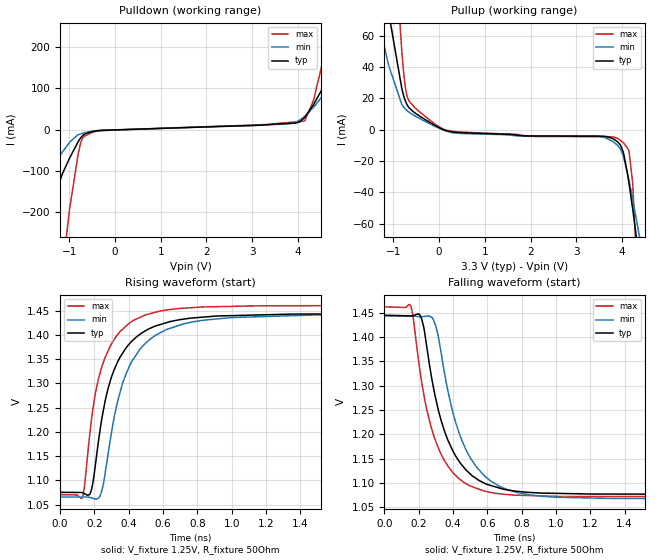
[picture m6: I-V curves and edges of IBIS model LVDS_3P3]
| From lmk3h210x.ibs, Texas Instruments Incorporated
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[Model]   LVDS_3P3
Model_type   Output
Polarity   Non-Inverting
Vmeas = 1.25
Vref = 1.25
Cref = 2pF
Rref = 50
|   typ   min   max
C_comp   2.5pF   2pF   3pF
[Voltage Range]   3.3   3.135   3.465
[Temperature Range]   45   125   -40
[Pullup Reference]   3.3   3.135   3.465
[Pulldown Reference]   -0   -0   0
[Power Clamp Reference]   3.3   3.135   3.465
[GND Clamp Reference]   0   0   0
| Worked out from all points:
|   slope of the pulldown table from 0 to 0.495 V, typ, clamps not added: 277 ohm
|   slope of the pullup table from 0 to 0.495 V, typ, clamps not added: 155 ohm
|   falling waveform, V_fixture 1.25V, R_fixture 50Ohm: 20-80 % time 175ps typ, 189ps min, 158ps max; typ from 1.45 V to 1.08 V
|   rising waveform, V_fixture 1.25V, R_fixture 50Ohm: 20-80 % time 169ps typ, 187ps min, 145ps max; typ from 1.08 V to 1.45 V
[Pulldown]
|   Voltage   I(typ)   I(min)   I(max)
-3.3V     -904.1mA   -523.3mA   -2.736A
-2.181V   -450.8mA   -243.4mA   -1.464A
-1.973V   -395.6mA   -197.8mA   -1.232A
-1.142V   -104.2mA   -52.74mA   -331.4mA
-815.1mV  -30.87mA   -12.56mA   -65.39mA
-706.2mV  -14.25mA   -8.667mA   -20.14mA
-379.5mV  -2.325mA   -1.992mA   -3.081mA
3.947V    16.26mA    18.26mA    18.71mA
4.343V    60.78mA    54.13mA    71.32mA
4.818V    154.5mA    120.5mA    290.7mA
5.531V    311.8mA    235mA      656.9mA
6.6V      565.9mA    436.6mA    1.236A
[Pullup]
|   Voltage   I(typ)   I(min)   I(max)
-3.3V     559.2mA    398.1mA    1.307A
-1.627V   181.2mA    113.3mA    436.1mA
-1.102V   74.25mA    40.77mA    176.2mA
-815.1mV  25.92mA    15.96mA    49.01mA
-706.2mV  16.12mA    12.31mA    21.86mA
125.4mV   -339.6uA   -524.8uA   5.45uA
3.482V    -4.055mA   -4.195mA   -4.389mA
3.907V    -7.84mA    -10.07mA   -5.625mA
4.026V    -14.21mA   -16.66mA   -8.257mA
4.155V    -34.39mA   -32.62mA   -13.98mA
4.363V    -79.27mA   -64.97mA   -112mA
6.6V      -897.2mA   -568.5mA   -2.5A
[Ramp]
R_load = 50
|   typ   min   max
dV/dt_r   0.221734/1.68524e-10   0.226535/1.86389e-10   0.234997/1.4465e-10
dV/dt_f   0.221734/1.74991e-10   0.226535/1.8778e-10   0.234997/1.57669e-10
[Falling Waveform]
V_fixture = 1.25V
V_fixture_min = 1.25V
V_fixture_max = 1.25V
R_fixture = 50Ohm
C_fixture = 0F
|   Time   V(typ)   V(min)   V(max)
0s        1.445V     1.444V     1.463V
155ps     1.444V     1.444V     1.463V
217.3ps   1.438V     1.442V     1.308V
279.6ps   1.309V     1.44V      1.207V
312.7ps   1.253V     1.405V     1.174V
350.7ps   1.207V     1.326V     1.146V
435.5ps   1.145V     1.203V     1.109V
584.2ps   1.099V     1.114V     1.083V
1ns       1.078V     1.07V      1.072V
5ns       1.076V     1.066V     1.071V
[Rising Waveform]
V_fixture = 1.25V
V_fixture_min = 1.25V
V_fixture_max = 1.25V
R_fixture = 50Ohm
C_fixture = 0F
|   Time   V(typ)   V(min)   V(max)
0s        1.076V     1.066V     1.071V
131.8ps   1.075V     1.066V     1.067V
178.6ps   1.076V     1.065V     1.214V
226.2ps   1.188V     1.064V     1.313V
250.9ps   1.243V     1.091V     1.343V
294.4ps   1.308V     1.188V     1.378V
381.5ps   1.372V     1.317V     1.417V
584.2ps   1.421V     1.404V     1.449V
1.47ns    1.443V     1.441V     1.46V
5ns       1.445V     1.444V     1.463V
